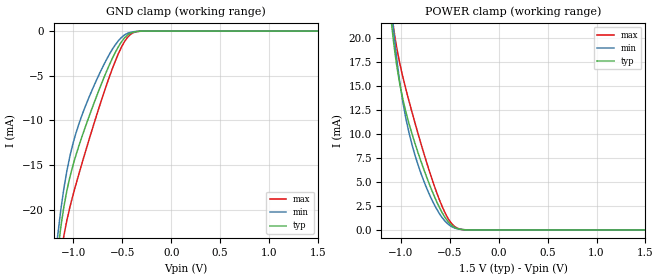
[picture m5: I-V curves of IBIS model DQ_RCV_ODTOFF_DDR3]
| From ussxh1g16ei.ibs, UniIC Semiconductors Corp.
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|   Model DQ_RCV_ODTOFF_DDR3
[Model] DQ_RCV_ODTOFF_DDR3
Model_type Input
Vinl =  0.615V
Vinh =  0.885V
C_comp   1.232pF   1.219pF   1.235pF
[Model Spec]
Vinh   0.885V   0.847V   0.922V
Vinl   0.615V   0.577V   0.652V
[Temperature Range]   25.000   95.000   -40.000
[Voltage Range]   1.500V   1.425V   1.575V
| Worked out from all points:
|   GND clamp passes 1 mA (typ) near -0.49 V on its own axis
|   POWER clamp passes 1 mA (typ) near -0.53 V on its own axis
[GND_clamp]
|Voltage   I(typ)   I(min)   I(max)
-1.5V     -77.15mA   -73.99mA   -84.26mA
-1.159V   -24.58mA   -22.75mA   -27.74mA
-1.128V   -21.88mA   -19.96mA   -25.03mA
-1.097V   -19.64mA   -17.59mA   -22.88mA
-1.066V   -17.82mA   -15.61mA   -21.14mA
-1.004V   -15mA      -12.58mA   -18.36mA
-880mV    -10.79mA   -8.48mA    -13.61mA
-632mV    -3.776mA   -2.594mA   -5.119mA
-477mV    -756.2uA   -431.9uA   -1.164mA
-415mV    -225.6uA   -131.2uA   -354.1uA
-322mV    -19.15uA   -14.82uA   -24.1uA
1.5V      0A         0A         0A
[POWER_clamp]
|Voltage   I(typ)   I(min)   I(max)
-1.5V     91.1mA     92.64mA    94.46mA
-1.104V   22.28mA    23.97mA    23.43mA
-1.073V   19.41mA    20.63mA    20.89mA
-1.042V   17.07mA    17.76mA    18.91mA
-980mV    13.62mA    13.3mA     15.93mA
-918mV    11.11mA    10.16mA    13.45mA
-856mV    9.013mA    7.787mA    11.15mA
-670mV    3.78mA     2.864mA    4.931mA
-577mV    1.775mA    1.269mA    2.414mA
-484mV    502.3uA    362.1uA    693.5uA
-329mV    12.96uA    15.92uA    9.805uA
1.5V      0A         0A         0A
